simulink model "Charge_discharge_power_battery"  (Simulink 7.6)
settings: Solver=ode23tb  StartTime=0.0  StopTime=N  MaxStep=0.1  RelTol=1e-4
InitFcn:
  | N=1800; % durée de la simulation
  | 
  | switch_on=80;
  | switch_off=40;
  | 
  | positive_SlewRate=80;
  | negative_SlewRate=-80;
  | 
  | negative_torque=-200;
StopFcn:
  | close all
  | load voltage_SOC.mat
  | plotyy(x(1,:),x(2,:),x(1,:),x(3,:))
  | axis([0 1800 180 300])
  | grid
  | title('Tension batterie (Volts) et état de charge (%)')
  | xlabel('temps')
  | 
  | figure
  | 
  | load couple_courant.mat
  | plotyy(y(1,:),y(2,:),y(1,:),y(3,:))
  | axis([0 1800 -210 10])
  | grid
  | title('Couple mécanique (Nm) et courant de batterie')
  | xlabel('temps')
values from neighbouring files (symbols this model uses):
  A = [1+j -(1-j);1 -2/(1-j)]    [systeme_AX_B_phaseurs.m]
undefined symbols (not defined in the file or in its folder): constant, Hydride, Metal, Nickel, Torque
libraries: powerlib x4, electricdrivelib x1

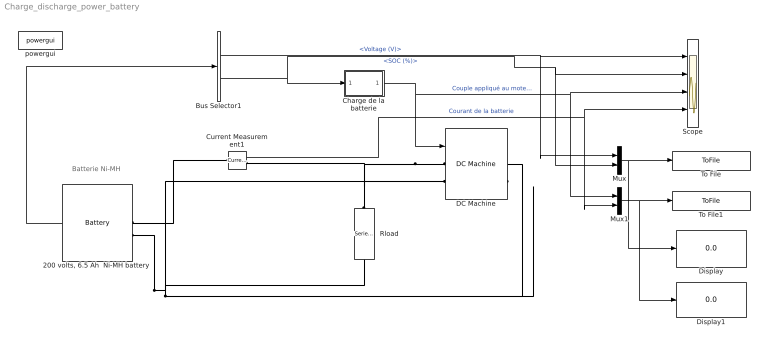
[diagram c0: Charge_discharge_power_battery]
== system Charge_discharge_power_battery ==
  note: Batterie Ni-MH
  " Rload" : powerlib/Elements/Series RLC Branch  DialogController=POWERSYS.PowerSysDialog  PhysicalDomain=powersysdomain  SubClassName=unknown  LeftPortType=p1  RightPortType=p1  LConnTagsString=__new0  RConnTagsString=__new0  BranchType=R  Resistance=10  Inductance=1e-3  SetiL0=off  InitialCurrent=0  Capacitance=1e-6  Setx0=off  InitialVoltage=0  Measurements=None
  "200 volts, 6.5 Ah  Ni-MH battery " : electricdrivelib/Extra Sources/Battery  DialogController=POWERSYS.PowerSysDialog  SystemSampleTime=-1  BatType=Nickel-Metal-Hydride  ShowDetailedParameters=off  NomV=200  NomQ=6.5  SOC=100  PresetModel=on  MaxQ=7  FullV=235.5932  Dis_rate=1.3  R=0.30769  Normal_OP=6.25  expZone="[216.9492           1.3]"  Dis_Char=off  current=50  Units=Ampere-hour  Batt_Tr=30
  Bus Selector1 : BusSelector  OutputSignals=Voltage (V),SOC (%)
  Charge de la batterie : Subsystem  mask{switch_on=switch_on, switch_off=switch_off, positive_SlewRate=positive_SlewRate, negative_SlewRate=negative_SlewRate, negative_torque=negative_torque}
      mask prompts: switch_on "Seuil de décharge batterie"; switch_off "Seuil de charge batterie"; positive_SlewRate "Slew rate1"; negative_SlewRate "SlewRate2"; negative_torque "Valeur du couple"
  Current Measurement1 : powerlib/Measurements/Current Measurement  DialogController=POWERSYS.PowerSysDialog  SystemSampleTime=-1  PhasorSimulation=off  OutputType=Complex  PSBequivalent=0
  DC Machine : powerlib/Machines/DC Machine  DialogController=POWERSYS.PowerSysDialog  SystemSampleTime=-1  PresetModel=No  MechanicalLoad=Torque TL  FieldType=Wound  ShowDetailedParameters=on  RLa=[0.4832 0.006763]  RLf=[84.91 13.39]  Laf=0.7096  MachineConstant=Torque constant (N.m/A)  Ke=1.8  Kt=1.8  J=0.2053  Bm=0.007032  Tf=0  w0=0  Ifinit=0  TsPowergui=0  TsBlock=-1
  Display : Display
  Display1 : Display
  Mux : Mux  Inputs=2
  Mux1 : Mux  Inputs=2
  Scope : Scope  NumInputPorts=4
  To File : ToFile  Filename=voltage_SOC  MatrixName=x
  To File1 : ToFile  Filename=couple_courant  MatrixName=y
  powergui : powerlib/powergui  SystemSampleTime=-1  SimulationMode=Continuous  SampleTime=0.001  frequency=60  SPID=off  DisableSnubberDevices=off  DisableRonSwitches=off  DisableVfSwitches=off  SwTol=0  Interpol=off  frequencyindice=0  echomessages=off  HookPort=off  DisplayEquations=off  FunctionMessages=off  EnableUseOfTLC=off  x0status=blocks  RestoreLinks=warning  ResistiveCurrentMeasurement=off  Frange=[0:2:500]  Ylog=off  Xlog=on  ShowGrid=off  save=off  variable=ZData  ZoomFFT=on  StartTime=0.0  cycles=1  DisplayStyle=1  fundamental=60  FreqAxis=off  MaxFrequency=1000  frequencyindicesteady=1  RmsSteady=1  display=off  Ts=0  methode=off
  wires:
  Charge de la batterie/1(s) -> DC Machine/1, Scope/3, Mux1/1  "Couple appliqué au moteur"
  "200 volts, 6.5 Ah  Ni-MH battery "/1 -> Bus Selector1/1
  Bus Selector1/2 -> Charge de la batterie/1(e), Scope/2, Mux/2  "<SOC (%)>"
  Bus Selector1/1 -> Scope/1, Mux/1  "<Voltage (V)>"
  Current Measurement1/1 -> Scope/4, Mux1/2  "Courant de la batterie"
  Mux/1 -> To File/1, Display/1
  Mux1/1 -> To File1/1, Display1/1
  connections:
  "200 volts, 6.5 Ah  Ni-MH battery "/LConn2 -- DC Machine/RConn1 -- DC Machine/RConn2 -- " Rload"/RConn1
  DC Machine/LConn2 -- DC Machine/LConn1 -- Current Measurement1/RConn1 -- " Rload"/LConn1
  Current Measurement1/LConn1 -- "200 volts, 6.5 Ah  Ni-MH battery "/LConn1

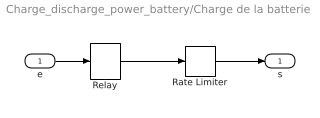
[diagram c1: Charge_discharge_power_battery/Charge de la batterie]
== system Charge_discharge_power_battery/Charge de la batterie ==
  e : Inport
  Rate Limiter : RateLimiter  RisingSlewLimit=positive_SlewRate  FallingSlewLimit=negative_SlewRate  SampleTimeMode=inherited
  Relay : Relay  OnSwitchValue=switch_on  OffSwitchValue=switch_off  OnOutputValue=0  OffOutputValue=negative_torque
  s : Outport
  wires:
  Rate Limiter/1 -> s/1
  e/1 -> Relay/1
  Relay/1 -> Rate Limiter/1
